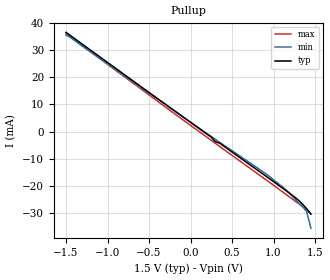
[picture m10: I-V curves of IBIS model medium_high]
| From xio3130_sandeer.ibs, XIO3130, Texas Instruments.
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|[Falling Waveform]
|R_fixture = 50
|V_fixture = 1.0V
|V_fixture_min = 0.9V
|V_fixture_max = 1.1V
|0.00000S   1.26200V   1.126200V   1.3900V
|10.00000pS   1.10000V   0.92880V   1.26100V
|20.00000pS   0.99720V   0.82760V   1.16100V
|30.00000pS   0.94260V   0.76770V   1.09600V
|40.00000pS   0.89460V   0.73400V   1.05700V
|50.00000pS   0.87190V   0.71010V   1.02700V
|60.00000pS   0.85170V   0.69790V   1.00900V
|70.00000pS   0.84070V   0.68820V   0.99620V
|80.00000pS   0.83070V   0.68150V   0.98750V
|90.00000pS   0.82470V   0.67590V   0.98040V
|0.10000nS   0.81920V   0.67150V   0.97570V
|0.11000nS   0.81570V   0.66790V   0.97190V
|0.12000nS   0.81250V   0.66490V   0.96930V
|0.13000nS   0.81030V   0.66240V   0.96700V
|0.14000nS   0.80840V   0.66040V   0.96550V
|0.15000nS   0.80700V   0.65860V   0.96420V
|0.16000nS   0.80570V   0.65720V   0.96320V
|0.17000nS   0.80480V   0.65590V   0.96230V
|0.18000nS   0.80400V   0.65490V   0.96170V
|0.19000nS   0.80340V   0.65390V   0.96120V
|0.20000nS   0.80280V   0.65310V   0.96070V
|0.21000nS   0.80230V   0.65240V   0.96030V
|0.22000nS   0.80190V   0.65180V   0.96000V
|0.23000nS   0.80160V   0.65130V   0.95970V
|0.24000nS   0.80120V   0.65080V   0.95950V
|0.25000nS   0.80100V   0.65040V   0.95920V
|0.26000nS   0.80070V   0.65000V   0.95910V
|0.27000nS   0.80050V   0.64970V   0.95890V
|0.28000nS   0.80040V   0.64940V   0.95870V
|0.29000nS   0.80020V   0.64920V   0.95860V
|0.30000nS   0.80000V   0.64890V   0.95840V
|0.31000nS   0.79990V   0.64870V   0.95830V
|0.32000nS   0.79980V   0.64850V   0.95820V
|0.33000nS   0.79960V   0.64840V   0.95810V
|0.34000nS   0.79950V   0.64820V   0.95800V
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[Model] medium_high
Model_type Open_source
Polarity Non-Inverting
Cref = 2.0pF
Rref = 50
Vref = 0.9V
Vmeas =1.0V
|   typ   min   max
C_comp   1.603pF   1.594pF   1.637pF
[Temperature Range]   25   125   -40
[Voltage Range] 1.50V 1.35V 1.65V
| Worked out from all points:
|   slope of the pullup table from 0 to 0.225 V, typ, clamps not added: 45.8 ohm
| (Process strength) nominal weak strong
[Pullup]
-1.5V     36.45mA    35.5mA     35.94mA
250mV     -2.021mA   -1.797mA   -3.18mA
300mV     -3.711mA   -2.83mA    -4.282mA
350mV     -4.199mA   -3.864mA   -5.386mA
950mV     -17.23mA   -16.42mA   -18.56mA
1.15V     -21.64mA   -21.3mA    -23mA
1.3V      -25.15mA   -26.16mA   -26.4mA
1.35V     -26.61mA   -27.4mA    -27.53mA
1.4V      -28.31mA   -29.4mA    -28.73mA
1.45V     -30.23mA   -35.4mA    -30.2mA
[Ramp]
| variable   typ   min   max
dV/dt_r 0.1938V/0.0411567ns  0.19662V/0.0449788ns  0.192V/0.0389468ns
|dV/dt_f 0.18726V/0.0374755ns  0.1902V/0.0346605ns  0.1854V/0.0369998ns
dV/dt_f 0.18726V/0.000374755ns  0.1902V/0.0346605ns  0.1854V/0.0369998ns
R_load = 50
